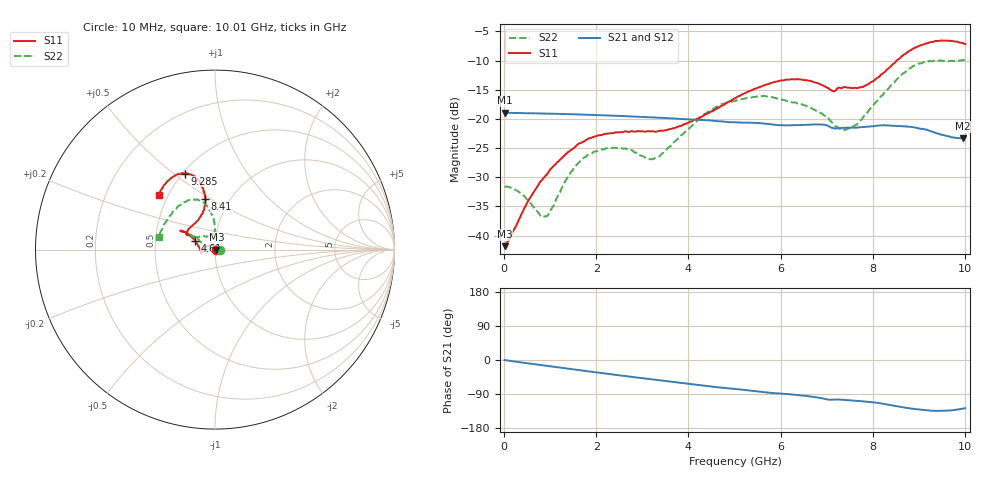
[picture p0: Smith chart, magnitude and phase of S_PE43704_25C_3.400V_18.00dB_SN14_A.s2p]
! Device ID: PE43704
! Dir: z:\PE43704\PE43704_Char_1_20130516\PE43704\AMB\3p400V\18p00dB
! Serial: 14
! Insertion: A
! Impedance: 50 ohm
! Temp: Amb
! VDD: 3.400V
! Attenuation Step: 18.00dB
! IDD: 1.140536e-01mA
#  Hz  S  RI  R  50
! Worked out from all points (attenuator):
!   401 points, 10 MHz to 10.01 GHz, reference 50 ohm
!   highest |S21| = -18.95 dB at 10 MHz (marker M1); lowest = -23.3 dB at 9.96 GHz (marker M2)
!   lowest |S11| = -41.8 dB at 10 MHz (marker M3), VSWR 1.02, Z = 50.8 + j0.0411 ohm
!   |S11| at or under -10 dB: start of sweep to 8.523 GHz
!   |S22| runs from -36.8 to -9.9 dB; largest |S21 - S12| = 0.0011
!   S11 on the Smith chart (normalised r, x): 10 MHz: 1.02, +0.00; 4.61 GHz: 0.79, +0.08; 8.41 GHz: 0.77, +0.48; 9.285 GHz: 0.51, +0.55; 10.01 GHz: 0.44, +0.34
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1e7  0.00812 0.000405  0.1128 -0.000393  0.1129 -0.00031  0.0261 0.000201
3.35e8  0.00395 0.0136  0.1117 -0.0111  0.1117 -0.0111  0.0212 0.00973
8.85e8  -0.0206 0.0247  0.1075 -0.0282  0.1074 -0.0282  -0.0032 0.0143
1.01e9  -0.0279 0.0246  0.1062 -0.0319  0.1062 -0.0319  -0.0108 0.0126
1.41e9  -0.0502 0.0158  0.1009 -0.0433  0.1009 -0.0433  -0.0333 0.000489
1.685e9  -0.0624 0.00675  0.0965 -0.0506  0.0966 -0.0506  -0.044 -0.0102
2.385e9  -0.0748 -0.0144  0.0832 -0.0665  0.0832 -0.0664  -0.0507 -0.0254
3.135e9  -0.0765 -0.0165  0.0663 -0.0795  0.0663 -0.0795  -0.0448 -0.00834
3.36e9  -0.0784 -0.0105  0.0608 -0.0824  0.0609 -0.0823  -0.0474 0.00176
4.61e9  -0.1121 0.0502  0.0302 -0.091  0.0306 -0.0908  -0.106 0.0694
5.01e9  -0.1318 0.0715  0.0219 -0.0909  0.0219 -0.0909  -0.1226 0.0732
5.96e9  -0.1832 0.1048  0.00281 -0.0885  0.00288 -0.0886  -0.1283 0.0742
6.685e9  -0.1839 0.1  -0.0109 -0.0887  -0.0109 -0.0887  -0.1013 0.069
7.135e9  -0.1508 0.0848  -0.0212 -0.0807  -0.021 -0.0808  -0.0541 0.073
7.46e9  -0.1397 0.1212  -0.0231 -0.0809  -0.0234 -0.0809  -0.0219 0.08
7.835e9  -0.0907 0.1704  -0.0288 -0.0804  -0.0287 -0.0804  -0.00176 0.1085
8.36e9  -0.0538 0.2695  -0.0419 -0.0771  -0.0418 -0.0773  -0.013 0.1854
8.41e9  -0.0543 0.2832  -0.0432 -0.076  -0.0431 -0.0762  -0.019 0.1953
8.86e9  -0.0921 0.3854  -0.053 -0.0666  -0.0526 -0.0667  -0.0756 0.2703
9.285e9  -0.1667 0.4235  -0.054 -0.0562  -0.0543 -0.056  -0.1599 0.2672
9.96e9  -0.3054 0.3243  -0.0425 -0.0535  -0.0429 -0.0537  -0.3069 0.0911
1.001e10  -0.3129 0.3061  -0.042 -0.0551  -0.0426 -0.0548  -0.3119 0.0697
